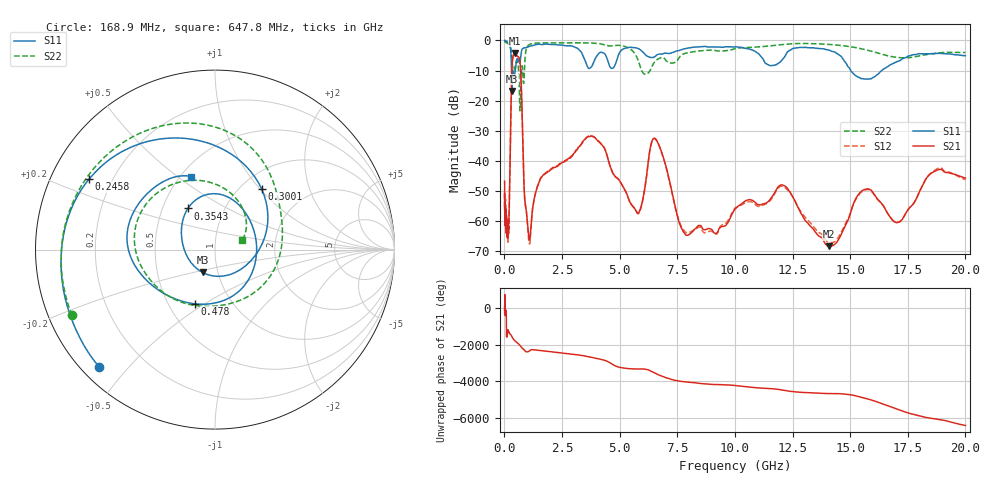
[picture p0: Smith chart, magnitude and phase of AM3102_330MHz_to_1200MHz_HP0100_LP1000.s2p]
! Date/Time: Tue, Sep 11, 2018 5:13 PM
! Network Analyzer: Agilent Technologies E8362B Rev: A.07.50.63
! Sweep from 0.010 to 20.000 GHz, 1601 Points, Sweep Type: LOG
! Power Supply: 4.950 V, 0.001 A
# Hz S DB R 50
!freq MagS11 AngS11 MagS21 AngS21 MagS12 AngS12 MagS22 AngS22
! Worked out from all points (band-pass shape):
!   1601 points, 10 MHz to 20 GHz, reference 50 ohm
!   highest |S21| = -4.15 dB at 445.1 MHz (marker M1); lowest = -68.4 dB at 14.07 GHz (marker M2)
!   |S21| within 3 dB of the highest: 342.9 MHz to 677.4 MHz (334.5 MHz wide, 65.6 % of centre)
!   lowest |S11| = -16.8 dB at 330 MHz (marker M3), VSWR 1.34, Z = 42.2 - j11 ohm
!   |S11| at or under -10 dB: 308.1 MHz to 475.4 MHz (167.4 MHz wide, 42.7 % of centre); 15.03 GHz to 16.37 GHz (1.348 GHz wide, 8.59 % of centre)
!   |S22| runs from -23.4 to -0.3 dB; largest |S21 - S12| = 0.012
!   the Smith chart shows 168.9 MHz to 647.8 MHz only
!   S11 on the Smith chart (normalised r, x): 168.9 MHz: 0.05, -0.42; 245.8 MHz: 0.12, +0.26; 300.1 MHz: 1.24, +1.02; 354.3 MHz: 0.67, +0.33; 478 MHz: 0.68, -0.46; 647.8 MHz: 0.57, +0.56
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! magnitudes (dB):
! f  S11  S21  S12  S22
! 10 MHz  0.0  -46.8  -50.8  -0.3
! 35.55 MHz  0.0  -58.1  -59.2  -0.5
! 126.4 MHz  -0.4  -64.1  -62.7  -0.9
! 168.9 MHz  -0.7  -62.4  -65.3  -1.1
! 245.8 MHz  -1.9  -41.1  -41.1  -1.9
! 300.1 MHz  -7.4  -16.8  -16.9  -3.7
! 330 MHz  -16.8  -8.7  -8.7  -6.6
! 354.3 MHz  -11.2  -6.3  -6.4  -8.4
! 445.1 MHz  -11.6  -4.2  -4.2  -9.2
! 447.2 MHz  -11.5  -4.2  -4.2  -9.1
! 478 MHz  -9.8  -4.2  -4.3  -8.2
! 647.8 MHz  -7.4  -5.9  -6.0  -15.8
! 873.8 MHz  -2.4  -51.6  -52.0  -9.3
! 1.072 GHz  -2.0  -66.2  -67.1  -1.4
! 1.59 GHz  -1.3  -45.6  -45.8  -0.8
! 3.793 GHz  -8.7  -31.8  -31.7  -0.9
! 5.652 GHz  -2.4  -55.9  -56.0  -4.3
! 6.58 GHz  -5.0  -32.9  -33.1  -6.6
! 7.882 GHz  -2.7  -64.8  -63.9  -4.2
! 12.09 GHz  -6.1  -48.2  -48.6  -1.3
! 14.07 GHz  -3.2  -68.4  -67.1  -1.3
! 20 GHz  -5.0  -45.8  -46.4  -4.0
